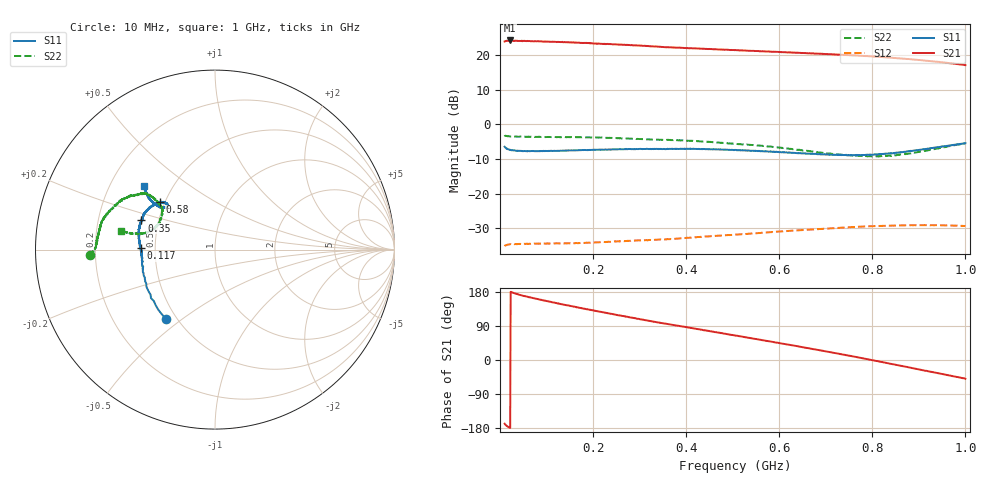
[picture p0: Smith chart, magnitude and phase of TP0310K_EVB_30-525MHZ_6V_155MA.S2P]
!Agilent Technologies,E5071C,MY46523237,B.13.01
!Date: Wed Aug 09 14:25:58 2023
!Data & Calibration Information:
!Freq	S11:SOLT2(ON)	S21:SOLT2(ON)	S12:SOLT2(ON)	S22:SOLT2(ON)
!PortZ  Port1:50+j0  Port2:50+j0
!Above PortZ is port z conversion or system Z0 setting when saving the data.
!When reading, reference impedance value at option line is always used.
# Hz S dB R 50
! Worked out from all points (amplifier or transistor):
!   991 points, 10 MHz to 1 GHz, reference 50 ohm
!   highest |S21| = 24.2 dB at 21 MHz (marker M1)
!   |S21| within 3 dB of that: start of sweep to 544.3 MHz
!   unconditionally stable (mu >= 1): start of sweep to end of sweep
!   at 175 MHz: K = 1.20, MAG = 26.2 dB, |S12| = -34.3 dB
!   at 505 MHz: K = 1.20, MAG = 23.9 dB, |S12| = -31.9 dB
!   at 1 GHz: K = 1.25, MAG = 20.2 dB, |S12| = -29.4 dB
!   S11 on the Smith chart (normalised r, x): 10 MHz: 0.44, -0.44; 117 MHz: 0.41, +0.01; 350 MHz: 0.40, +0.16; 580 MHz: 0.47, +0.30; 1 GHz: 0.34, +0.34
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1e7  -6.48 -125.0  23.88 -168.0  -35.18 27.7  -3.13 -177.5
2.1e7  -7.39 -153.7  24.18 -178.7  -34.65 12.5  -3.48 179.7
3.1e7  -7.55 -163.6  24.04 176.4  -34.61 7.4  -3.55 178.4
5e7  -7.77 -171.1  24.06 169.3  -34.51 3.0  -3.59 176.8
8.7e7  -7.70 -177.8  23.91 159.1  -34.40 -0.7  -3.66 173.6
1.17e8  -7.66 179.0  23.81 151.5  -34.41 -2.5  -3.68 170.9
1.75e8  -7.47 174.3  23.49 136.8  -34.25 -6.3  -3.74 166.5
2.11e8  -7.37 170.6  23.24 128.2  -34.09 -8.9  -3.81 164.0
2.52e8  -7.27 167.5  23.04 118.7  -33.77 -10.9  -4.04 161.0
3e8  -7.11 163.1  22.73 107.8  -33.52 -13.6  -4.28 157.0
3.4e8  -7.11 159.3  22.39 99.1  -33.32 -16.6  -4.45 154.1
3.5e8  -7.11 158.4  22.33 96.9  -33.23 -17.7  -4.50 153.4
4.24e8  -7.16 151.9  21.88 81.7  -32.55 -22.9  -4.90 149.3
5.05e8  -7.39 144.5  21.40 64.9  -31.86 -30.3  -5.64 143.8
5.8e8  -7.86 139.3  20.97 48.8  -31.14 -39.0  -6.40 140.6
6.7e8  -8.53 136.5  20.46 29.5  -30.38 -50.0  -7.86 140.7
7.14e8  -8.81 136.6  20.17 19.5  -30.01 -56.6  -8.54 142.0
7.64e8  -8.89 138.4  19.86 8.2  -29.63 -64.5  -9.10 147.2
8.35e8  -8.50 141.9  19.23 -8.9  -29.27 -76.5  -9.10 158.7
9.11e8  -7.17 142.5  18.42 -27.4  -29.09 -90.7  -7.76 167.2
9.62e8  -6.20 140.9  17.69 -40.0  -29.19 -100.2  -6.41 169.0
1e9  -5.45 138.2  17.07 -49.5  -29.40 -107.5  -5.47 168.6
